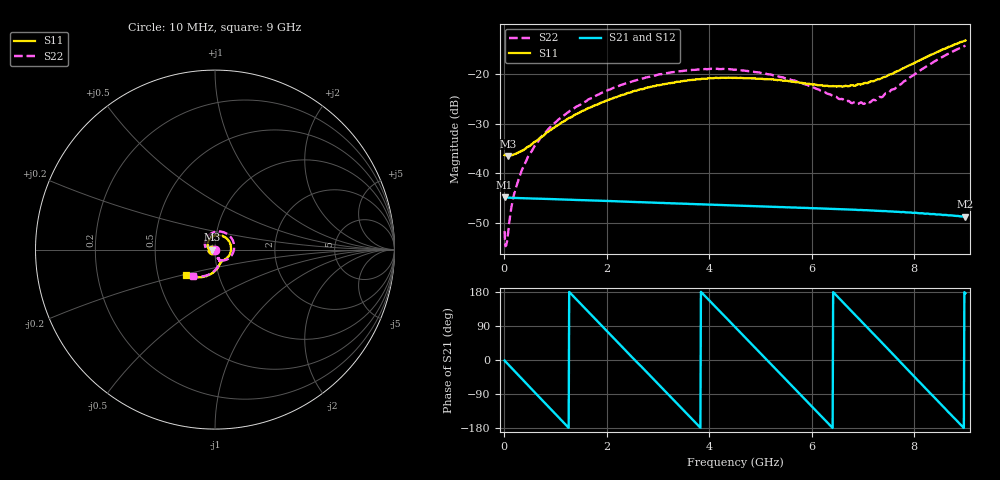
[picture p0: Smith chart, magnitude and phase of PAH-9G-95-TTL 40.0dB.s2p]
! MTS Systemtechnik GmbH
! S-Parameters
! Model: PAH-9G/95-TTL
! Attenuation Step: 40.0dB
#  HZ  S  DB  R  50.00
! Rohde & Schwarz Vector Network Analyzer
! Rohde-Schwarz,ZNB20-2Port,1334333062101652,3.45
! Created: UTC 1/26/2024, 7:21:35 AM
! freq[Hz]  db:S11  ang:S11  db:S21  ang:S21  db:S12  ang:S12  db:S22  ang:S22
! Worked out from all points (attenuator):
!   900 points, 10 MHz to 9 GHz, reference 50 ohm
!   highest |S21| = -44.82 dB at 10 MHz (marker M1); lowest = -48.7 dB at 9 GHz (marker M2)
!   lowest |S11| = -36.5 dB at 80 MHz (marker M3), VSWR 1.03, Z = 48.5 - j0.0905 ohm
!   |S11| at or under -10 dB: start of sweep to end of sweep
!   |S22| runs from -54.6 to -14.4 dB; largest |S21 - S12| = 0.00017
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1e7  -36.33 -171.6  -44.82 -1.4  -44.83 -1.4  -51.60 -113.7
5e7  -36.41 -176.7  -44.87 -7.4  -44.90 -7.4  -54.08 -120.1
8e7  -36.50 -176.4  -44.89 -11.7  -44.92 -11.7  -51.80 -111.5
1.5e8  -36.36 -174.6  -44.92 -21.8  -44.96 -21.8  -46.37 -109.4
2.1e8  -36.16 -173.4  -44.94 -30.4  -44.97 -30.4  -43.61 -108.6
3.3e8  -35.55 -170.3  -44.98 -47.4  -45.02 -47.4  -39.78 -114.8
4.8e8  -34.60 -169.1  -45.03 -68.8  -45.08 -68.7  -36.42 -122.7
7.2e8  -32.78 -171.8  -45.11 -102.7  -45.14 -102.6  -32.73 -137.8
9.1e8  -31.31 -176.8  -45.17 -129.6  -45.20 -129.5  -30.62 -149.5
1.51e9  -27.54 161.1  -45.38 145.9  -45.41 146.1  -25.98 174.2
2.14e9  -24.85 132.4  -45.60 57.6  -45.62 57.6  -22.81 138.6
3.01e9  -22.30 92.1  -45.92 -64.1  -45.95 -64.1  -20.17 92.0
3.78e9  -21.11 55.4  -46.20 -171.7  -46.23 -171.4  -19.16 52.3
4.51e9  -20.83 21.2  -46.46 86.5  -46.49 86.9  -19.17 15.2
5.31e9  -21.26 -15.3  -46.74 -25.5  -46.78 -24.7  -20.40 -24.9
6.01e9  -22.16 -42.6  -47.00 -123.5  -47.03 -122.3  -22.63 -55.6
6.54e9  -22.48 -58.2  -47.19 162.2  -47.25 163.5  -25.08 -70.3
6.9e9  -22.14 -65.7  -47.36 111.8  -47.38 113.1  -26.07 -71.0
7.15e9  -21.56 -70.1  -47.47 76.8  -47.49 77.9  -25.69 -68.6
7.51e9  -20.21 -78.6  -47.65 26.2  -47.67 27.2  -23.77 -68.2
8.24e9  -16.65 -104.2  -48.10 -77.0  -48.15 -75.5  -18.51 -91.5
9e9  -13.31 -138.9  -48.71 176.2  -48.78 177.9  -14.35 -128.9
